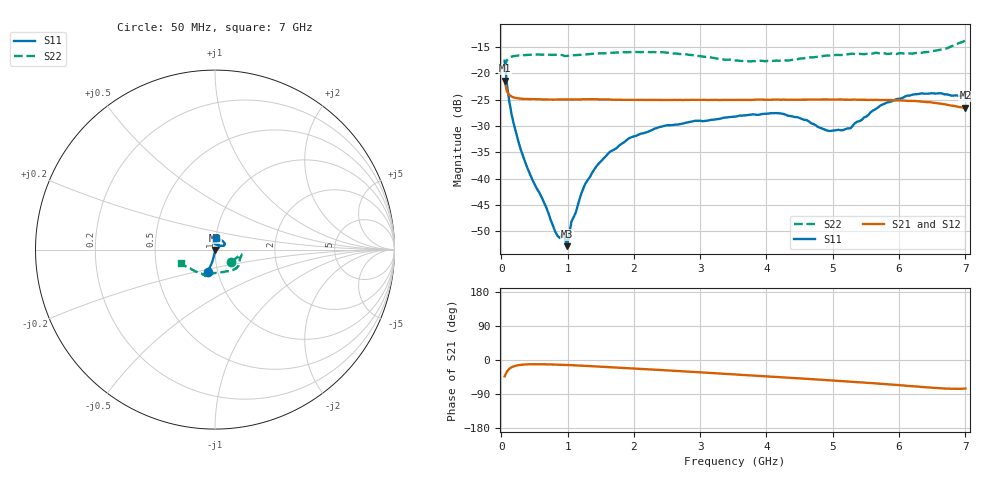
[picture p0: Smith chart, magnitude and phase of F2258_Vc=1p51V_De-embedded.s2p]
! Integrated Device Technology
! Corporate Headquarters
! 6024 Silver Creek Valley Road
! San Jose, CA 95138  USA
! Phone:  1-408-284-8200
! Toll Free:  1-800-223-1366
! Webpage:  http://www.idt.com/
! Timing and RF Division
! 515 Groton Road, Suite 102
! Westford, MA 01886-6024
! Device:  F2258
! Description: Voltage Variable RF Attenuator
! Frequency:  50.0 -  6000.00 MHz
! Package:  3x3 mm Thin QFN Plastic Package: 16 pin
! Ports:  2 RF, 2 DC
!  Pin  1  = NC
!  Pin  2  = NC
!  Pin  3  = RF2  = Port 2
!  Pin  4  = GND
!  Pin  5  = Vdd
!  Pin  6  = NC
!  Pin  7  = VCTRL
!  Pin  8  = NC
!  Pin  9  = GND
!  Pin 10  = RF1  = Port 1
!  Pin 11  = NC
!  Pin 12  = NC
!  Pin 13  = NC
!  Pin 14  = NC
!  Pin 15  = NC
!  Pin 16  = NC
! Vcntrl:  1.510 Volts
! Vdd:  +3.300 Volts
! Current:  1.161 mA
! Data:  The device was measured on a the F2258 evaluation board which has
!  individual transmission lines to the RF pins.  Data was collected
!  using a calibrated network analyzer.  The evaluation board was
!  de-embedded using a TRL calibration technique.
!  The reference plane is the edge of the package pin.
! Misc:  SN 10
!  Action Tracker AT0285
! Date Measured:  2014-12-10
! Date:  2016-01-13  MJV
! Note:
!  Integrated Device Technology supplies this data as a sample of measured
!  data at the package pin for this product.  Your particular data for this
!  product may vary.
!  Data was taken at 25 degrees C.
!  Integrated Device Technology reserves the right to change this data at anytime.
!Freq_(GHz)  S11M_(dB)  S11P_(deg)  S21M_(dB)  S21P_(deg)  S12M_(dB)  S12P_(deg)  S22M_(dB)  S22P_(deg)
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# GHz S dB R 50
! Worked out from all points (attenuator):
!   201 points, 50 MHz to 7 GHz, reference 50 ohm
!   highest |S21| = -21.42 dB at 50 MHz (marker M1); lowest = -26.6 dB at 7 GHz (marker M2)
!   lowest |S11| = -52.8 dB at 988.2 MHz (marker M3), VSWR 1.00, Z = 50.1 - j0.184 ohm
!   |S11| at or under -10 dB: start of sweep to end of sweep
!   |S22| runs from -18.9 to -13.8 dB; largest |S21 - S12| = 0.00053
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0.05  -17.63 -108.3  -21.42 -43.2  -21.40 -43.2  -18.88 -36.2
0.08475  -22.10 -103.5  -23.45 -30.5  -23.41 -30.5  -17.54 -17.9
0.15425  -27.77 -100.7  -24.44 -19.3  -24.43 -19.3  -16.86 -11.0
0.29325  -34.50 -97.8  -24.83 -12.8  -24.79 -12.8  -16.61 -9.4
0.8145  -50.10 -46.7  -25.01 -12.1  -24.96 -12.1  -16.53 -16.3
0.884  -51.31 -16.2  -24.97 -12.5  -24.97 -12.5  -16.55 -17.9
0.9535  -50.91 -68.7  -24.97 -13.0  -24.98 -13.0  -16.74 -18.5
0.98825  -52.84 -53.6  -24.97 -13.2  -24.96 -13.2  -16.74 -19.5
1.05775  -48.18 -14.6  -24.99 -13.7  -24.96 -13.7  -16.63 -20.6
1.2315  -42.05 9.0  -24.96 -15.1  -24.93 -15.1  -16.46 -23.6
1.44  -37.57 14.0  -24.96 -17.2  -24.98 -17.2  -16.28 -27.0
1.6485  -34.84 18.6  -25.02 -19.2  -24.99 -19.2  -16.13 -30.3
1.9265  -32.36 27.2  -25.08 -21.8  -25.02 -21.8  -16.00 -34.5
2.37825  -30.26 38.6  -25.09 -26.2  -25.04 -26.2  -16.04 -41.8
3.525  -28.25 87.2  -25.06 -38.0  -25.01 -38.1  -17.58 -70.8
4.1505  -27.57 103.3  -25.01 -44.8  -25.04 -44.8  -17.59 -91.7
4.7065  -29.64 93.5  -25.00 -50.8  -24.98 -50.8  -17.00 -103.7
4.94975  -30.98 76.0  -25.01 -53.5  -24.99 -53.5  -16.66 -106.5
5.2625  -30.49 47.5  -25.04 -57.1  -25.08 -57.0  -16.33 -107.8
5.85325  -25.47 25.5  -25.10 -64.5  -25.15 -64.5  -16.32 -112.0
6.33975  -23.81 31.8  -25.40 -71.2  -25.41 -71.2  -16.15 -124.4
7  -24.00 83.6  -26.56 -75.4  -26.51 -75.4  -13.79 -158.0
